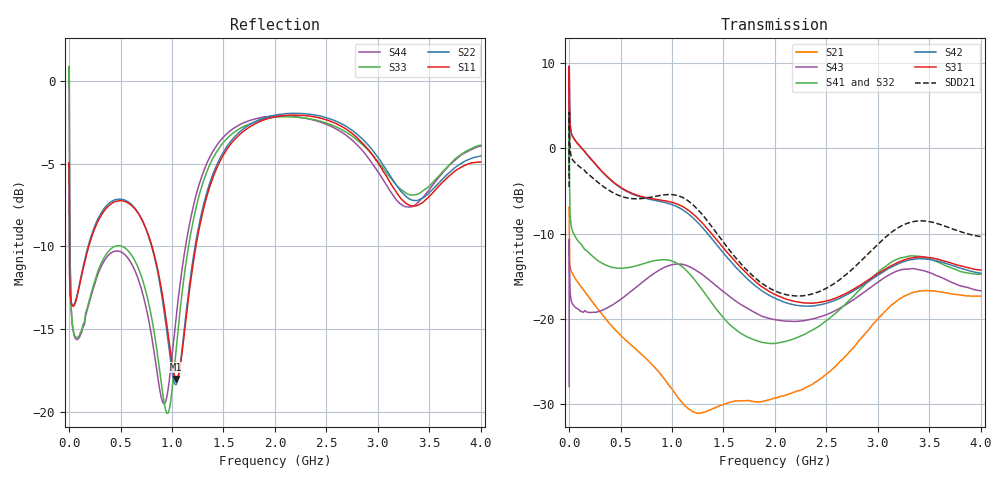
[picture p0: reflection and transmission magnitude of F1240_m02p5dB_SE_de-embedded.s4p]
! Integrated Device Technology
! Corporate Headquarters
! 6024 Silver Creek Valley Road
! San Jose, CA 95138  USA
! Phone:  1-408-284-8200
! Toll Free:  1-800-223-1366
! Webpage:  http://www.idt.com/
! Timing and RF Division
! 515 Groton Road, Suite 102
! Westford, MA 01886-6024
! Device:  F1240
! Description: Dual Intermediate Frequency Digital Variable Gain Amplifier
! Frequency:  10.0 -  500.00 MHz
! Package:  5x5 mm QFN Plastic Package: 32 pin
! Ports:  8 RF, 20 DC
!  Pin  1  = GA3 / Data  Pin 17  = RF OUT_B+
!  Pin  2  = GA4 / CLK  Pin 18  = RF OUT_B-
!  Pin  3  = GA5  Pin 19  = STBY_B
!  Pin  4  = VMODE  Pin 20  = Ground
!  Pin  5  = No Connect  Pin 21  = Ground
!  Pin  6  = GB5  Pin 22  = STB_A
!  Pin  7  = GB4  Pin 23  = RF OUT_A-  = Port 4
!  Pin  8  = GB3  Pin 24  = RF OUT_A+  = Port 3
!  Pin  9  = GB2  Pin 25  = GA0
!  Pin 10  = GB1  Pin 26  = ISET_A
!  Pin 11  = RF IN_B+  Pin 27  = VCC
!  Pin 12  = RF IN_B-  Pin 28  = Ground
!  Pin 13  = Ground  Pin 29  = RF IN_A-  = Port 2
!  Pin 14  = VCC  Pin 30  = RF IN_A+  = Port 1
!  Pin 15  = ISET_B  Pin 31  = GA1
!  Pin 16  = GB0  Pin 32  = GA2 / CSb
! Gain  = +19.5 dB
! State  = 1
! Voltage  = +5.00 V
! Current  = 85.292 mA (one channel only)
! Temperture  =  +25 C
! Test Date  =  2017-10-18
! Board  =  EB4031
! Data:  The device was measured on a custom evaluation board which has
!  individual transmission lines to the RF pins.  Data was collected
!  using a calibrated network analyzer.  The evaluation board was
!  de-embedded using Automatic Fixture Removal.
!  The reference plane is the edge of the package pin.
!  Only Channel A was measured.
!  This data is in single-ended operation.  If your needs are balanced
!  or differential S-parameters then this file needs to be used a
!  linear simulator.
! File Date:  2017-11-10  MJV
! Note:
!  Integrated Device Technology supplies this data as a sample of measured
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# Hz S dB R 100
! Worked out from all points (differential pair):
!   410 points, 500 kHz to 4 GHz, reference 100 ohm
!   strongest paths, dB at 500 kHz, 930 MHz, 1.96 GHz, 2.98 GHz, 4 GHz:
!     S31: 2.2, -6.1, -16.9, -14.9, -14.3
!     S42: 2.2, -6.4, -17.4, -15.1, -14.7
!     S41: -3.1, -13.1, -22.9, -14.8, -14.8
!     S32: -3.1, -13.3, -22.9, -15.1, -15.2
!     S43: -28.0, -14.0, -20.0, -15.9, -16.7
!     S21: -7.0, -27.1, -29.5, -20.3, -17.3
!   taken as a pair (ports 1,2 in; 3,4 out), SDD21 dB: -4.5, -5.5, -16.5, -11.5, -10.4
!   lowest |S11| = -18.0 dB at 1.04 GHz (marker M1), VSWR 1.29, Z = 78.8 - j7.54 ohm
!   |S11| at or under -10 dB: 3.245 MHz to 191.6 MHz (188.4 MHz wide, 193 % of centre); 805.6 MHz to 1.232 GHz (426.7 MHz wide, 41.9 % of centre)
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500000  -5.16 -5.6  -7.03 -5.8  -30.63 79.7  -35.84 77.8
        -7.04 -5.8  -5.15 -5.6  -35.79 76.6  -30.61 80.9
        2.21 -108.6  -3.11 -111.1  -0.22 0.5  -27.99 -41.6
        -3.14 -110.0  2.21 -107.5  -27.99 -41.6  -0.23 2.8
2000000  -7.26 -34.3  -9.72 -34.0  -21.47 27.4  -27.53 7.2
         -9.73 -34.0  -7.23 -34.4  -27.48 6.9  -21.45 27.7
         9.32 -177.4  3.27 163.1  -0.06 -50.7  -10.67 -141.0
         3.22 163.4  9.33 -177.1  -10.66 -141.0  -0.11 -50.4
4000000  -10.94 -32.7  -13.12 -24.1  -21.85 8.0  -30.70 -13.6
         -13.12 -24.1  -10.93 -33.1  -30.67 -13.8  -21.84 8.2
         6.10 159.6  -2.79 137.5  -4.56 -84.3  -13.23 174.8
         -2.84 137.7  6.11 159.8  -13.22 174.7  -4.61 -84.3
1.7e8  -10.50 -100.9  -17.10 -55.3  -24.30 -42.9  -35.45 -34.9
       -17.11 -55.2  -10.35 -102.3  -35.51 -34.7  -24.31 -43.2
       -0.66 117.1  -12.03 87.7  -13.87 -152.0  -19.23 108.6
       -12.01 87.5  -0.65 116.2  -19.20 108.1  -14.00 -152.1
1.04e9  -18.02 -158.0  -29.42 159.8  -24.17 151.9  -31.87 -169.1
        -28.96 159.4  -18.37 -154.4  -31.83 -164.3  -24.88 151.4
        -6.49 -92.6  -13.62 172.2  -16.20 -111.0  -13.78 -130.1
        -13.43 167.9  -6.80 -95.2  -13.59 -130.1  -14.28 -108.1
2.86e9  -3.84 97.3  -22.05 -26.8  -25.28 -150.0  -27.57 -134.3
        -21.98 -26.7  -3.59 98.3  -28.39 -122.2  -26.45 -144.5
        -15.84 -62.8  -16.53 -148.9  -3.92 102.4  -17.83 -82.2
        -16.18 -159.4  -16.02 -59.8  -16.95 -79.6  -4.29 95.4
4e9  -4.90 -141.7  -17.38 106.2  -23.64 -37.5  -24.72 -22.0
     -17.34 106.2  -4.55 -139.8  -25.70 -6.9  -25.35 -30.7
     -14.30 45.7  -15.24 -57.1  -3.89 -133.7  -18.30 65.7
     -14.77 -70.1  -14.67 51.6  -16.72 57.5  -3.94 -143.5
